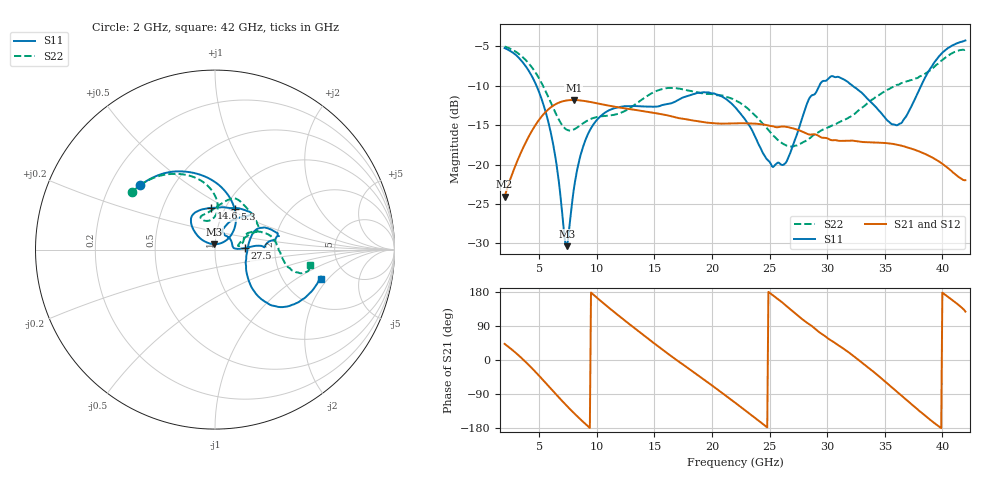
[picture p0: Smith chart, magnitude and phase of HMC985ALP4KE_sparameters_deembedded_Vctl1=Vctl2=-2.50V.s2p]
!s2p File: Measurements: S11, S21, S12, S22
# GHz S dB R 50.0
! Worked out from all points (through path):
!   401 points, 2 GHz to 42 GHz, reference 50 ohm
!   highest |S21| = -11.79 dB at 8 GHz (marker M1); lowest = -24.1 dB at 2 GHz (marker M2)
!   lowest |S11| = -30.3 dB at 7.4 GHz (marker M3), VSWR 1.06, Z = 49.6 + j3 ohm
!   |S11| at or under -10 dB: 4.772 GHz to 29.31 GHz (24.54 GHz wide, 144 % of centre); 32.21 GHz to 38.15 GHz (5.93 GHz wide, 16.9 % of centre)
!   |S22| runs from -17.7 to -5.0 dB; largest |S21 - S12| = 0.00032
!   S11 on the Smith chart (normalised r, x): 2 GHz: 0.33, +0.34; 5.3 GHz: 1.11, +0.53; 14.6 GHz: 0.86, +0.42; 27.5 GHz: 1.40, +0.02; 42 GHz: 3.24, -1.68
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2  -5.21 139.2  -24.07 42.5  -24.08 42.5  -5.01 145.3
3.6  -7.06 105.5  -17.88 1.4  -17.89 1.4  -6.40 118.1
5.3  -12.06 63.9  -13.73 -51.6  -13.73 -51.7  -9.90 91.9
6.3  -18.11 42.4  -12.44 -85.2  -12.44 -85.2  -13.05 86.4
7.4  -30.34 96.5  -11.85 -121.0  -11.85 -121.0  -15.56 97.9
8  -23.20 140.9  -11.79 -139.5  -11.80 -139.5  -15.54 107.0
8.7  -18.25 141.6  -11.87 -160.0  -11.88 -160.0  -14.87 113.1
9.9  -14.52 133.9  -12.18 167.3  -12.19 167.3  -14.00 113.5
11.8  -12.73 122.3  -12.71 119.5  -12.71 119.5  -13.57 101.3
14.6  -12.64 95.0  -13.33 52.9  -13.33 52.9  -11.08 77.0
15.4  -12.59 85.2  -13.55 34.4  -13.55 34.4  -10.53 72.3
19.2  -10.82 45.4  -14.60 -49.4  -14.60 -49.4  -10.94 43.6
22  -12.69 51.0  -14.76 -112.4  -14.77 -112.4  -11.81 24.1
25.3  -20.30 55.4  -15.13 170.4  -15.13 170.4  -16.28 17.9
26.4  -19.78 6.1  -15.19 144.1  -15.19 144.0  -17.53 11.5
27.5  -15.60 2.7  -15.61 116.1  -15.61 116.0  -17.45 8.3
28.7  -11.18 2.6  -16.16 88.9  -16.17 88.8  -16.38 11.8
31.1  -8.94 15.2  -16.98 36.3  -16.99 36.3  -14.58 25.5
35.4  -14.59 6.5  -17.30 -66.4  -17.30 -66.4  -10.39 16.8
36.6  -14.38 -25.9  -17.65 -97.8  -17.65 -97.8  -9.62 10.7
39.4  -6.84 -43.6  -19.33 -168.6  -19.33 -168.6  -7.42 -13.8
42  -4.24 -15.2  -21.97 127.8  -21.98 127.8  -5.39 -9.2
